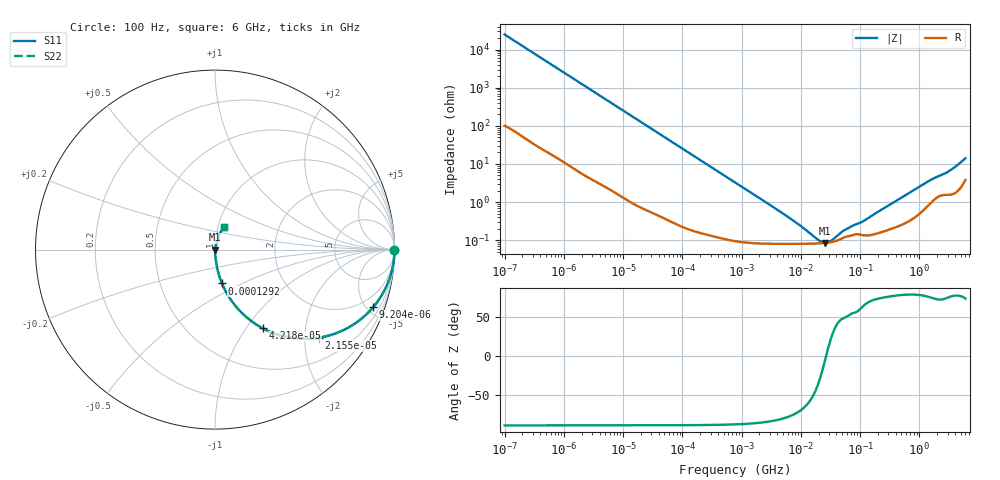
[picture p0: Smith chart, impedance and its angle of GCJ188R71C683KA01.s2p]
!Murata Part Number: GCJ188R71C683KA01
!These Parameters are Measured in Series Mode Connection
!Data Generated on Mar 13, 2026
!  o--ll--o
!Port1  Port2
!  o------o
!Operation Temp=25[degC], DC Bias Voltage=0[V]
!Freq. Start=100[Hz] Stop=6[GHz] 401[Steps]
# Hz S RI R 50
!Freq.(Hz) S11(Real) S11(Imag) S21(Real) S21(Imag) S12(Real) S12(Imag) S22(Real) S22(Imag)
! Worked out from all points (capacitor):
!   401 points, 100 Hz to 6 GHz, reference 50 ohm
!   read as one part in series: C = 63.9 nF near 109 Hz
!   lowest |Z| = 85.2 mohm at 25.46 MHz (marker M1)
!   series resonance near 26.73 MHz, so ESL is about 560 pH
!   S11 on the Smith chart (normalised r, x): 100 Hz: open; 9.204 kHz: 1.03, -5.48; 21.55 kHz: 1.01, -2.35; 42.18 kHz: 1.01, -1.20; 129.2 kHz: 1.00, -0.39; 6 GHz: 1.08, +0.27
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100  1 -0.00402  3.24e-05 0.00402  3.24e-05 0.00402  1 -0.00402
2008  0.9933 -0.0795  0.00671 0.0795  0.00671 0.0795  0.9933 -0.0795
4918  0.9623 -0.1879  0.0377 0.1879  0.0377 0.1879  0.9623 -0.1879
9204  0.8811 -0.3211  0.1189 0.3211  0.1189 0.3211  0.8811 -0.3211
21550  0.5785 -0.4909  0.4215 0.4909  0.4215 0.4909  0.5785 -0.4909
40335  0.2841 -0.4475  0.7159 0.4475  0.7159 0.4475  0.2841 -0.4475
42182  0.2665 -0.4386  0.7335 0.4386  0.7335 0.4386  0.2665 -0.4386
69028  0.121 -0.3222  0.879 0.3222  0.879 0.3222  0.121 -0.3222
129199  0.039 -0.1888  0.961 0.1888  0.961 0.1888  0.039 -0.1888
289253  0.00902 -0.0873  0.991 0.0873  0.991 0.0873  0.00902 -0.0873
774597  0.00203 -0.033  0.998 0.033  0.998 0.033  0.00203 -0.033
5809218  0.000817 -0.00421  0.9992 0.00421  0.9992 0.00421  0.000817 -0.00421
1.555665e7  0.000813 -0.00109  0.9992 0.00109  0.9992 0.00109  0.000813 -0.00109
2.128304e7  0.000829 -0.000444  0.9992 0.000444  0.9992 0.000444  0.000829 -0.000444
2.545746e7  0.000846 -9.4e-05  0.9992 9.4e-05  0.9992 9.4e-05  0.000846 -9.4e-05
3.184506e7  0.000884 0.000343  0.9991 -0.000343  0.9991 -0.000343  0.000884 0.000343
5.449875e7  0.0012 0.00139  0.9988 -0.00139  0.9988 -0.00139  0.0012 0.00139
1.115611e8  0.00136 0.00279  0.9986 -0.00279  0.9986 -0.00279  0.00136 0.00279
3.124326e8  0.00197 0.00817  0.998 -0.00817  0.998 -0.00817  0.00197 0.00817
1.431855e9  0.00938 0.0339  0.9906 -0.0339  0.9906 -0.0339  0.00938 0.0339
3.065283e9  0.0187 0.0587  0.9813 -0.0587  0.9813 -0.0587  0.0187 0.0587
6e9  0.0528 0.124  0.9472 -0.124  0.9472 -0.124  0.0528 0.124
